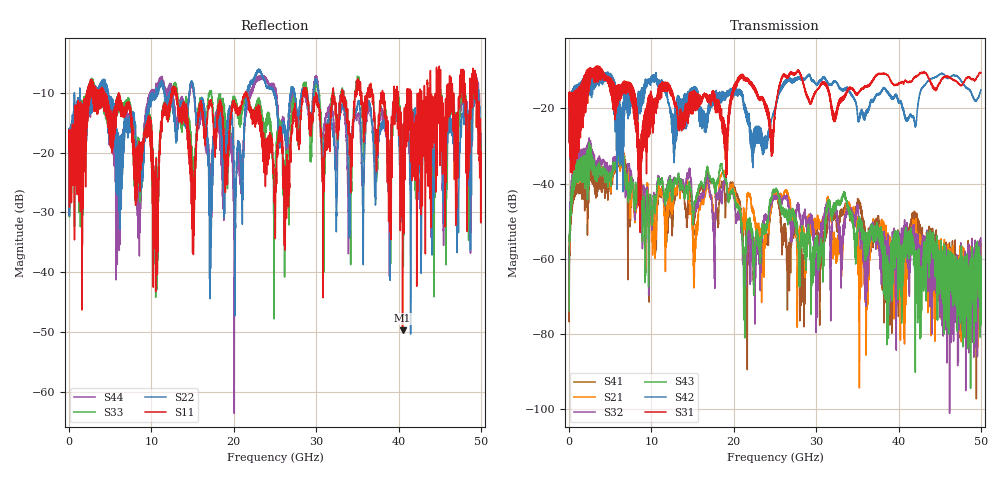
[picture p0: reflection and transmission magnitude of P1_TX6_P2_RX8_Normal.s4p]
!Keysight Technologies,N5225B,MY57041031,A.13.20.10
!Date: Friday, May 31, 2019 11:40:38
!Correction: S11(Full 4 Port(1,2,3,4))
!S12(Full 4 Port(1,2,3,4))
!S13(Full 4 Port(1,2,3,4))
!S14(Full 4 Port(1,2,3,4))
!S21(Full 4 Port(1,2,3,4))
!S22(Full 4 Port(1,2,3,4))
!S23(Full 4 Port(1,2,3,4))
!S24(Full 4 Port(1,2,3,4))
!S31(Full 4 Port(1,2,3,4))
!S32(Full 4 Port(1,2,3,4))
!S33(Full 4 Port(1,2,3,4))
!S34(Full 4 Port(1,2,3,4))
!S41(Full 4 Port(1,2,3,4))
!S42(Full 4 Port(1,2,3,4))
!S43(Full 4 Port(1,2,3,4))
!S44(Full 4 Port(1,2,3,4))
!S4P File: Measurements: <S11,S12,S13,S14>,
!<S21,S22,S23,S24>,
!<S31,S32,S33,S34>,
!<S41,S42,S43,S44>:
# Hz S  dB  R 50.0
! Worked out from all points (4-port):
!   5000 points, 10 MHz to 50 GHz, reference 50 ohm
!   strongest paths, dB at 10 MHz, 12.51 GHz, 25.01 GHz, 37.51 GHz, 50 GHz:
!     S31: -19.4, -15.5, -21.6, -10.8, -10.6
!     S42: -19.6, -22.2, -20.1, -16.4, -15.0
!     S43: -73.9, -43.0, -41.7, -52.0, -69.0
!     S32: -69.5, -41.5, -43.5, -54.4, -66.3
!     S21: -65.0, -46.8, -42.3, -57.3, -69.9
!     S41: -59.8, -49.0, -42.8, -49.7, -61.0
!   lowest |S11| = -49.7 dB at 40.49 GHz (marker M1), VSWR 1.01, Z = 50 - j0.324 ohm
!   |S11| at or under -10 dB: 4.287 GHz to 12.47 GHz (8.179 GHz wide, 97.6 % of centre); 13.02 GHz to 21.41 GHz (8.386 GHz wide, 48.7 % of centre); 21.57 GHz to 28.42 GHz (6.844 GHz wide, 27.4 % of centre)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
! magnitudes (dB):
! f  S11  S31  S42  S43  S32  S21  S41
! 10 MHz  -19.4  -19.4  -19.6  -73.9  -69.5  -65.0  -59.8
! 960 MHz  -17.3  -19.4  -17.6  -34.6  -32.3  -34.4  -36.8
! 6.34 GHz  -13.7  -16.6  -28.5  -31.4  -31.7  -31.8  -31.4
! 18.51 GHz  -12.2  -20.2  -16.5  -34.9  -44.2  -37.4  -39.9
! 21.3 GHz  -10.4  -12.4  -19.0  -63.3  -66.3  -48.9  -47.5
! 40.49 GHz  -49.7  -12.9  -20.0  -64.4  -56.6  -68.4  -63.0
! 50 GHz  -19.8  -10.6  -15.0  -69.0  -66.3  -69.9  -61.0
